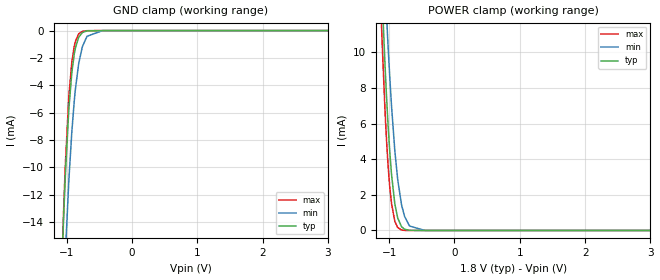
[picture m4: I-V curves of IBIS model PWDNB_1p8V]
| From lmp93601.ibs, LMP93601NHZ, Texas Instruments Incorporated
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|   Model PWDNB_1p8V
[Model]   PWDNB_1p8V
Model_type   Input
Vinl = 0.495
Vinh = 1.365
|   typ   min   max
|   (nom PVT)   (fast PVT)   (slow PVT)
C_comp   0.1436pF   0.1360pF   0.1525pF
[Model spec]
|subparameter
Vinl   0.54   0.495   0.585
Vinh   1.26   1.155   1.365
[Voltage Range]   1.8   1.65   1.95
[Temperature Range]   27   125   -25
[Power Clamp Reference]   1.8   1.65   1.95
[GND Clamp Reference]   0   0   0
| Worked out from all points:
|   GND clamp passes 1 mA (typ) near -0.85 V on its own axis
|   POWER clamp passes 1 mA (typ) near -0.89 V on its own axis
[GND Clamp]
|   Voltage   I(typ)   I(min)   I(max)
-1.8V     -170.4mA   -156.4mA   -184.9mA
-1.098V   -21.07mA   -26.31mA   -21.23mA
-1.049V   -14.24mA   -19.93mA   -13.71mA
-1.017V   -10.43mA   -16.14mA   -9.612mA
-968.4mV  -5.991mA   -11.25mA   -5.055mA
-919.8mV  -3.083mA   -7.399mA   -2.301mA
-865.8mV  -1.291mA   -4.321mA   -802.7uA
-817.2mV  -518.8uA   -2.495mA   -264.2uA
-757.8mV  -139.9uA   -1.171mA   -54.24uA
-687.6mV  -21.56uA   -417.6uA   -5.433uA
-450mV    -4.592nA   -2.822uA   0A
3.595V    0A         0A         0A
[POWER Clamp]
|   Voltage   I(typ)   I(min)   I(max)
-1.8V     102.5mA    97.39mA    106.2mA
-1.114V   13.89mA    18.33mA    11.33mA
-1.103V   12.87mA    17.37mA    10.29mA
-1.066V   9.567mA    14.16mA    6.998mA
-1.039V   7.489mA    12.04mA    5.04mA
-1.022V   6.37mA     10.84mA    4.041mA
-990mV    4.443mA    8.638mA    2.453mA
-909mV    1.433mA    4.347mA    489uA
-811.8mV  227uA      1.495mA    28.83uA
-687.6mV  7.321uA    250.8uA    174.7nA
-450mV    129.3pA    1.291uA    0A
3.595V    0A         0A         0A
